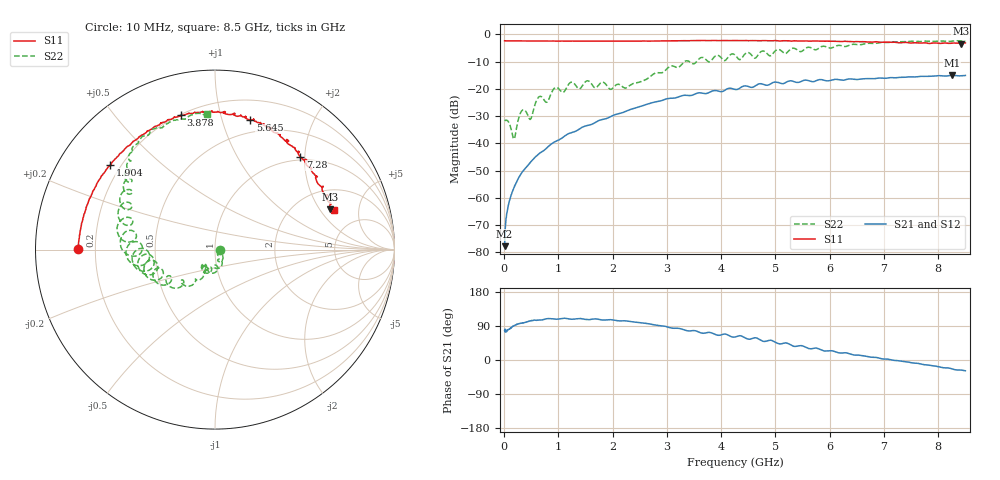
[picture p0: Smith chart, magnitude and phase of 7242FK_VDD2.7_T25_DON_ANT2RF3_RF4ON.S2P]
!Agilent Technologies,E5071C,MY46417908,A.11.23
!Date: Wed Dec 09 15:40:03 2020
!Data & Calibration Information:
!Freq	S11:SOLT2(ON)	S21:SOLT2(ON)	S12:SOLT2(ON)	S22:SOLT2(ON)
!PortZ  Port1:50+j0  Port2:50+j0
!Above PortZ is port z conversion or system Z0 setting when saving the data.
!When reading, reference impedance value at option line is always used.
# Hz S dB R 50
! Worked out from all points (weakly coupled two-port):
!   1601 points, 10 MHz to 8.5 GHz, reference 50 ohm
!   highest |S21| = -15.01 dB at 8.251 GHz (marker M1); lowest = -77.8 dB at 10 MHz (marker M2)
!   lowest |S11| = -3.4 dB at 8.415 GHz (marker M3), VSWR 5.20, Z = 150 + j124 ohm
!   |S11| at or under -10 dB: nowhere
!   |S22| runs from -38.4 to -2.3 dB; largest |S21 - S12| = 0.0023
!   S11 on the Smith chart (normalised r, x): 10 MHz: 0.13, +0.00; 1.904 GHz: 0.16, +0.35; 3.878 GHz: 0.20, +0.76; 5.645 GHz: 0.38, +1.24; 7.28 GHz: 0.94, +1.91; 8.5 GHz: 3.16, +2.71
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1e7  -2.33 179.7  -77.77 78.0  -77.18 85.3  -31.69 -2.7
7.898125e7  -2.37 178.2  -62.74 80.6  -62.82 79.1  -32.07 -32.7
1.851062e8  -2.39 175.9  -56.19 90.7  -56.14 90.5  -38.41 -25.2
3.336812e8  -2.40 172.9  -50.55 97.2  -50.62 97.6  -27.92 -34.7
4.822562e8  -2.42 169.8  -47.04 103.3  -47.07 103.3  -31.18 -51.4
6.4675e8  -2.43 166.6  -43.80 105.2  -43.79 105.4  -22.86 -57.7
7.900188e8  -2.45 163.7  -41.63 109.1  -41.65 109.0  -24.91 -68.0
9.332875e8  -2.45 161.0  -39.47 107.8  -39.46 108.1  -19.66 -74.8
1.235744e9  -2.45 154.6  -36.09 107.6  -36.09 107.7  -17.57 -95.8
1.426769e9  -2.45 150.9  -34.25 109.2  -34.25 109.1  -19.33 -99.7
1.904331e9  -2.50 141.1  -30.76 106.0  -30.76 106.0  -19.10 -130.1
2.843538e9  -2.43 121.2  -24.58 91.0  -24.59 91.0  -14.07 -123.0
3.878256e9  -2.24 104.1  -20.62 68.3  -20.63 68.3  -8.18 -154.4
4.255e9  -2.26 97.8  -20.21 60.7  -20.21 60.6  -7.58 -174.3
4.971344e9  -2.29 85.7  -17.56 48.9  -17.56 48.7  -6.61 -175.6
5.645238e9  -2.52 74.7  -17.18 29.5  -17.12 29.6  -4.82 153.4
5.671769e9  -2.46 73.6  -17.34 29.9  -17.28 29.8  -5.08 151.7
7.088538e9  -2.88 51.6  -15.94 1.7  -16.00 1.6  -2.97 129.9
7.279562e9  -3.07 47.3  -15.80 -2.2  -15.80 -2.4  -2.70 126.7
8.250606e9  -3.22 22.4  -15.01 -23.3  -15.08 -23.3  -2.47 101.7
8.4151e9  -3.39 19.4  -15.20 -26.5  -15.27 -26.7  -2.42 95.0
8.5e9  -3.12 18.4  -15.08 -28.5  -15.16 -28.4  -2.41 93.3
